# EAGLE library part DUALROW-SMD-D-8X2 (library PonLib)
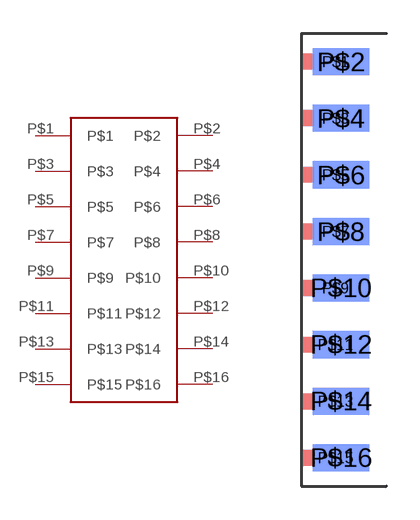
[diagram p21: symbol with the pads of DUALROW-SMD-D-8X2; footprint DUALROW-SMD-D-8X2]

Designator prefix -

## DUALROW-SMD-D-8X2  [DUALROW-SMD-D-8X2]
P$1  P$1
P$2  P$2
P$3  P$3
P$4  P$4
P$5  P$5
P$6  P$6
P$7  P$7
P$8  P$8
P$9  P$9
P$10  P$10
P$11  P$11
P$12  P$12
P$13  P$13
P$14  P$14
P$15  P$15
P$16  P$16

## Footprint DUALROW-SMD-D-8X2 (pad centres in mm)
smd 3.048 x 0.711: P$1 1.524,8.89; P$3 1.524,6.35; P$5 1.524,3.81; P$7 1.524,1.27; P$9 1.524,-1.27; P$11 1.524,-3.81; P$13 1.524,-6.35; P$15 1.524,-8.89
smd 2.54 x 1.219 bottom: P$2 1.778,8.89; P$4 1.778,6.35; P$6 1.778,3.81; P$8 1.778,1.27; P$10 1.778,-1.27; P$12 1.778,-3.81; P$14 1.778,-6.35; P$16 1.778,-8.89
